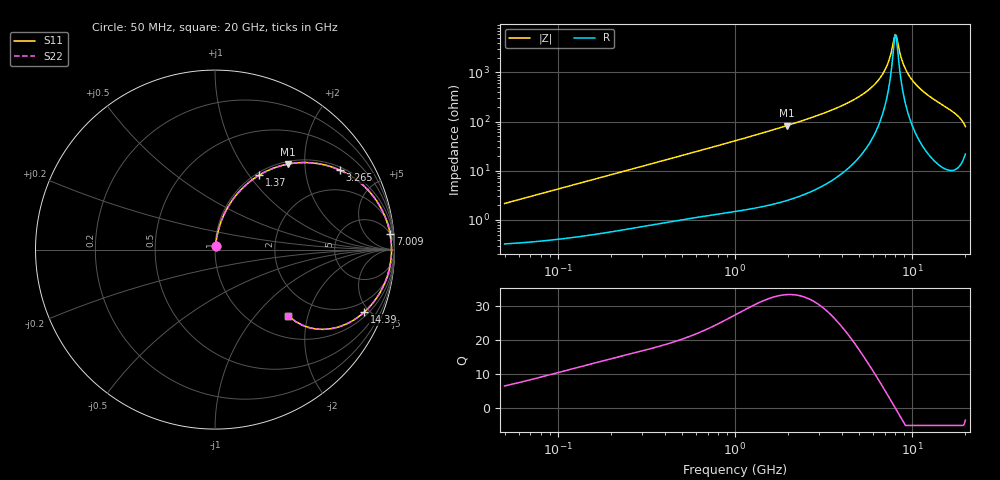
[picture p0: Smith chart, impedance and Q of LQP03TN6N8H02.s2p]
!Murata Part Number: LQP03TN6N8H02
!These Parameters are Measured in Series Mode Connection
!  o--[Z]--o
!Port1  Port2
!  o-------o
!Freq. Start=50[MHz] Stop=20[GHz], 401[Steps]
# Hz S RI R 50
!Freq.(Hz) S11(Real) S11(Imag) S21(Real) S21(Imag) S12(Real) S12(Imag) S22(Real) S22(Imag)
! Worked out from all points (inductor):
!   401 points, 50 MHz to 20 GHz, reference 50 ohm
!   read as one part in series: L = 6.78 nH near 51.52 MHz
!   highest Q = 33.3 at 1.962 GHz (marker M1), where L = 6.69 nH
!   self-resonance near 8.021 GHz
!   S11 on the Smith chart (normalised r, x): 50 MHz: 1.01, +0.04; 1.37 GHz: 1.04, +1.12; 3.265 GHz: 1.11, +3.08; 7.009 GHz: 5, +22; 14.39 GHz: 1.25, -4.66; 20 GHz: 1.44, -1.51
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5e7  0.00369 0.0212  0.9963 -0.0212  0.9963 -0.0212  0.00369 0.0212
1.364002e8  0.00785 0.0565  0.9922 -0.0565  0.9922 -0.0565  0.00785 0.0565
3.721004e8  0.0304 0.1463  0.9696 -0.1463  0.9696 -0.1463  0.0304 0.1463
1e9  0.1498 0.3391  0.8502 -0.3391  0.8502 -0.3391  0.1498 0.3391
1.369645e9  0.2457 0.4146  0.7543 -0.4146  0.7543 -0.4146  0.2457 0.4146
1.962148e9  0.4078 0.4766  0.5922 -0.4766  0.5922 -0.4766  0.4078 0.4766
2.728004e9  0.5935 0.4756  0.4065 -0.4756  0.4065 -0.4756  0.5935 0.4756
3.265178e9  0.6968 0.4426  0.3032 -0.4426  0.3032 -0.4426  0.6968 0.4426
4.275624e9  0.8342 0.35  0.1658 -0.35  0.1658 -0.35  0.8342 0.35
5.352748e9  0.9194 0.241  0.0806 -0.241  0.0806 -0.241  0.9194 0.241
6.311513e9  0.9603 0.1485  0.0397 -0.1485  0.0397 -0.1485  0.9603 0.1485
7.009217e9  0.9759 0.086  0.0241 -0.086  0.0241 -0.086  0.9759 0.086
7.442007e9  0.9811 0.0495  0.0189 -0.0495  0.0189 -0.0495  0.9811 0.0495
7.901521e9  0.9834 0.0125  0.0166 -0.0125  0.0166 -0.0125  0.9834 0.0125
8.141811e9  0.9836 -0.0061  0.0164 0.0061  0.0164 0.0061  0.9836 -0.0061
8.907419e9  0.9796 -0.0621  0.0204 0.0621  0.0204 0.0621  0.9796 -0.0621
9.892087e9  0.9664 -0.1274  0.0336 0.1274  0.0336 0.1274  0.9664 -0.1274
1.149051e10  0.9307 -0.2191  0.0693 0.2191  0.0693 0.2191  0.9307 -0.2191
1.438523e10  0.8322 -0.3478  0.1678 0.3478  0.1678 0.3478  0.8322 -0.3478
1.747767e10  0.6688 -0.436  0.3312 0.436  0.3312 0.436  0.6688 -0.436
1.88369e10  0.5522 -0.4406  0.4478 0.4406  0.4478 0.4406  0.5522 -0.4406
2e10  0.4078 -0.3677  0.5922 0.3677  0.5922 0.3677  0.4078 -0.3677
